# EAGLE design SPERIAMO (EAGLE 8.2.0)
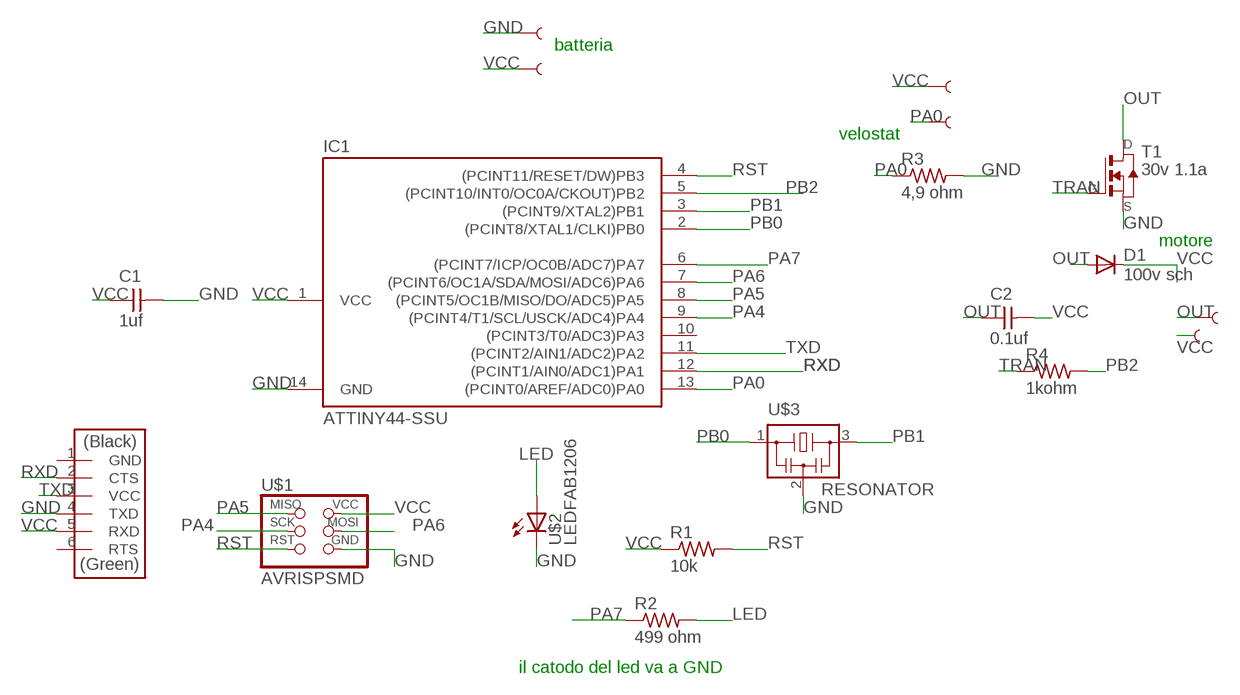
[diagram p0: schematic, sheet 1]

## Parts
C1  1uf  CAP-UNPOLARIZEDFAB  [C1206FAB]
C2  0.1uf  CAP-UNPOLARIZEDFAB  [C1206FAB]
D1  100v sch  DIODESOD123  [SOD123]
IC1  ATTINY44-SSU  [SOIC14]
R1  10k  RES-US1206FAB  [R1206FAB]
R2  499 ohm  RES-US1206FAB  [R1206FAB]
R3  4,9 ohm  RES-US1206FAB  [R1206FAB]
R4  1kohm  RES-US1206FAB  [R1206FAB]
T1  30v 1.1a  NMOSFETSOT23  [SOT-23]
U$1  AVRISPSMD  [2X03SMD]
U$2  LEDFAB1206  [LED1206FAB]
U$3  RESONATOR  [EFOBM]
U$4  FTDI-SMD-HEADER  [1X06SMD]
U$5  SEWTAP2  [PETAL-LONG-2]
U$6  SEWTAP2  [PETAL-LONG-2]
U$7  SEWTAP6  [PETAL-SMALL-2SIDE]
U$8  SEWTAP6  [PETAL-SMALL-2SIDE]
U$9  SEWTAP4  [PETAL-SMALL]
U$10  SEWTAP4  [PETAL-SMALL]

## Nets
GND: C1.2 IC1.14(GND) R3.2 T1.2(S) U$1.6(GND) U$2.2(C) U$3.2 U$4.4(TXD) U$10.1
LED: R2.2 U$2.1(A)
OUT: C2.1 D1.ANODE(A) T1.1(D) U$7.1
PA0: IC1.13((PCINT0/AREF/ADC0)PA0) R3.1 U$6.1
PA4: IC1.9((PCINT4/T1/SCL/USCK/ADC4)PA4) U$1.3(SCK)
PA5: IC1.8((PCINT5/OC1B/MISO/DO/ADC5)PA5) U$1.1(MISO)
PA6: IC1.7((PCINT6/OC1A/SDA/MOSI/ADC6)PA6) U$1.4(MOSI)
PA7: IC1.6((PCINT7/ICP/OC0B/ADC7)PA7) R2.1
PB0: IC1.2((PCINT8/XTAL1/CLKI)PB0) U$3.1
PB1: IC1.3((PCINT9/XTAL2)PB1) U$3.3
PB2: IC1.5((PCINT10/INT0/OC0A/CKOUT)PB2) R4.2
RST: IC1.4((PCINT11/RESET/DW)PB3) R1.2 U$1.5(RST)
RXD: IC1.12((PCINT1/AIN0/ADC1)PA1) U$4.2(CTS)
TRAN: R4.1 T1.3(G)
TXD: IC1.11((PCINT2/AIN1/ADC2)PA2) U$4.3(VCC)
VCC: C1.1 C2.2 D1.CATHODE(C) IC1.1(VCC) R1.1 U$1.2(VCC) U$4.5(RXD) U$5.1 U$8.1 U$9.1
Unconnected: IC1.10((PCINT3/T0/ADC3)PA3) U$4.1(GND) U$4.6(RTS)

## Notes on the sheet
- batteria
- velostat
- motore
- il catodo del led va a GND

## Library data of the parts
C1 C2 = 00_fab:CAP-UNPOLARIZED
D1 = 00_fab:DIODE: DIODE
IC1 = 00_fab:ATTINY44
R1-R4 = 00_fab:RES-US: Resistor (US Symbol)
T1 = 00_fab:NMOSFET: MOS FET
U$1 = 00_fab:AVRISP
U$2 = 00_fab:LED: LED
U$3 = 00_fab:RESONATOR
U$4 = 00_fab:FTDI-SMD-HEADER
U$5-U$10 = LilyPad-Wearables:SEWTAP

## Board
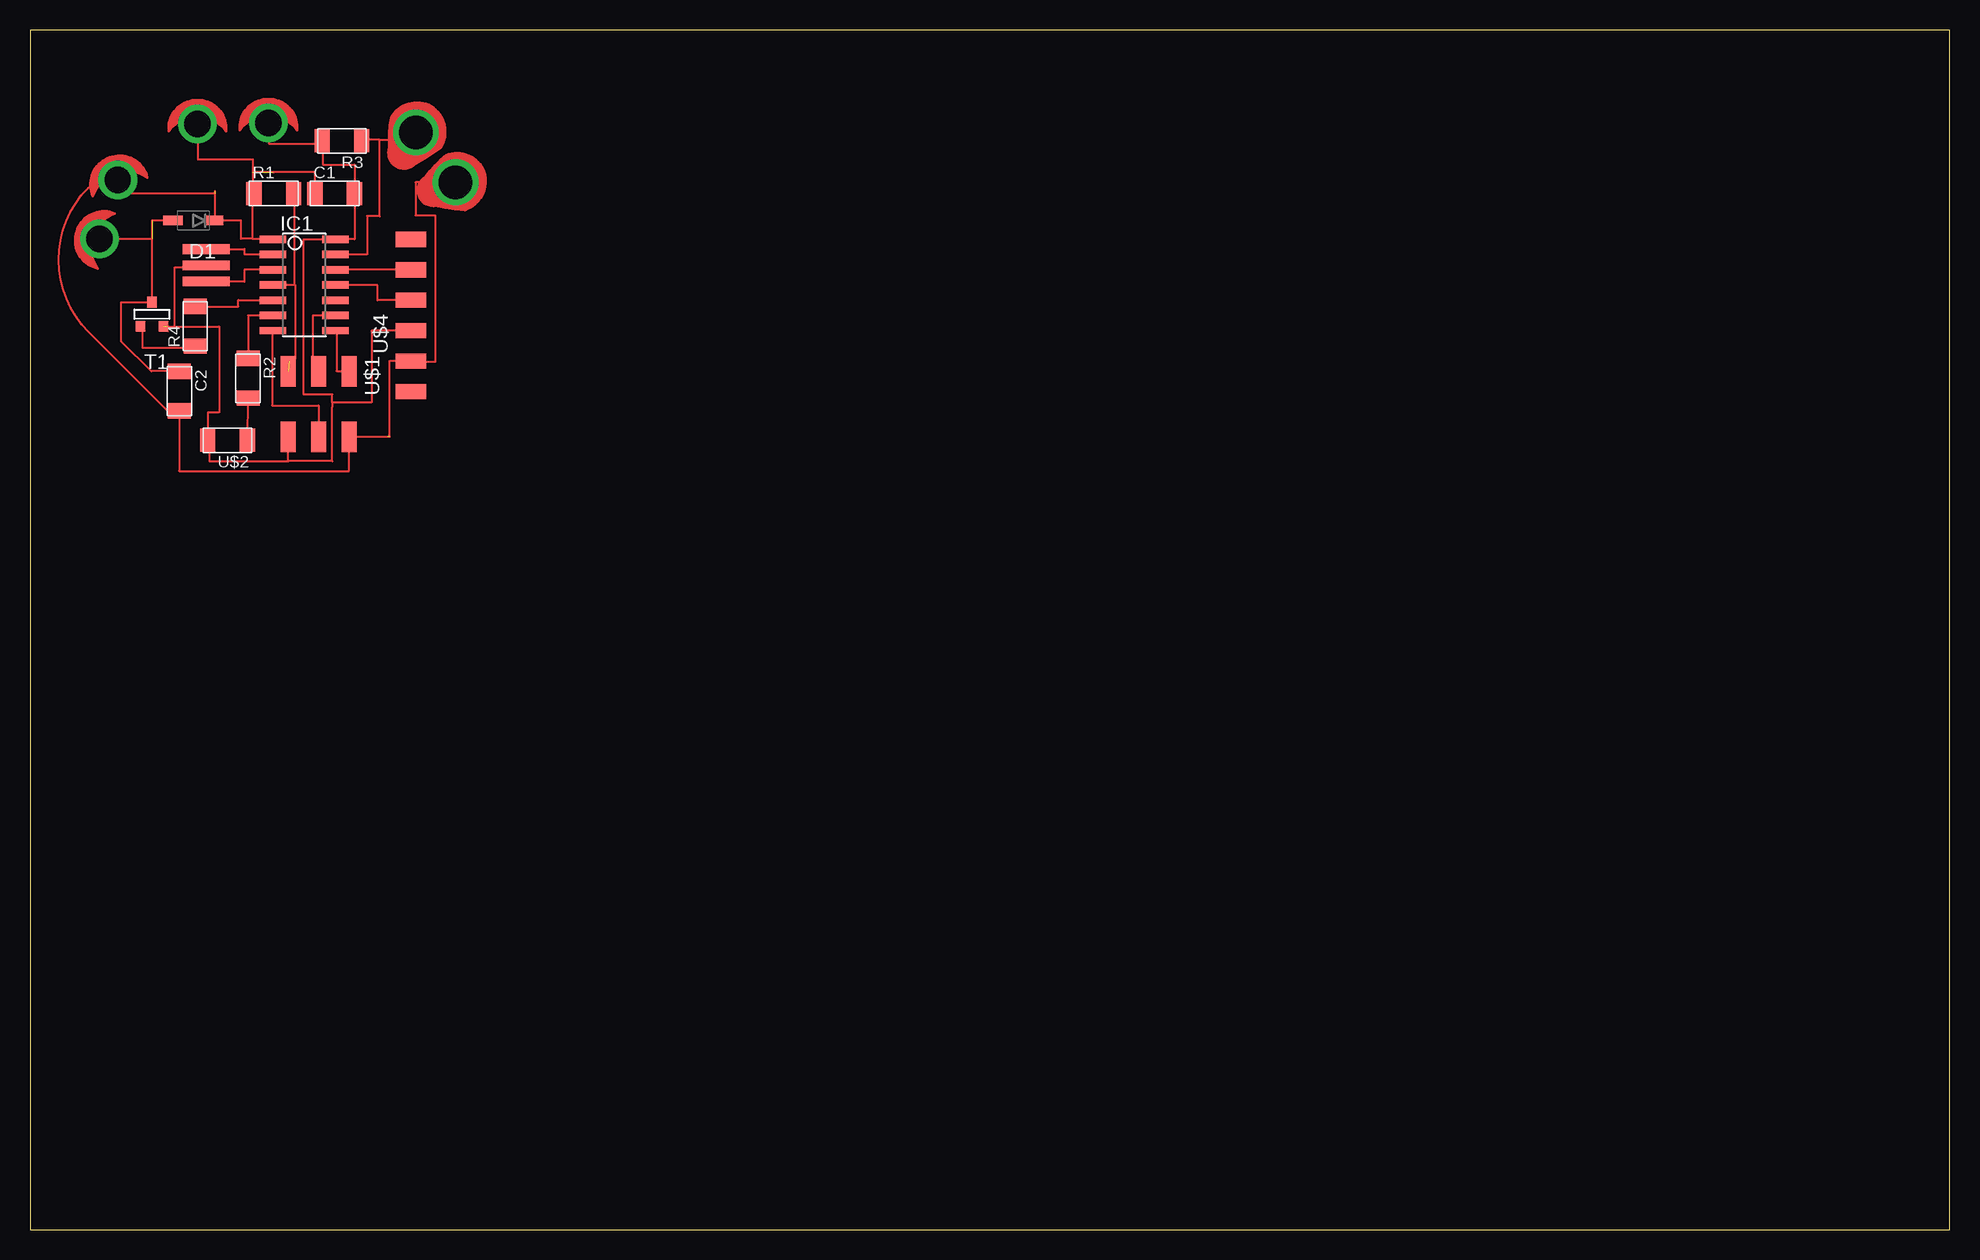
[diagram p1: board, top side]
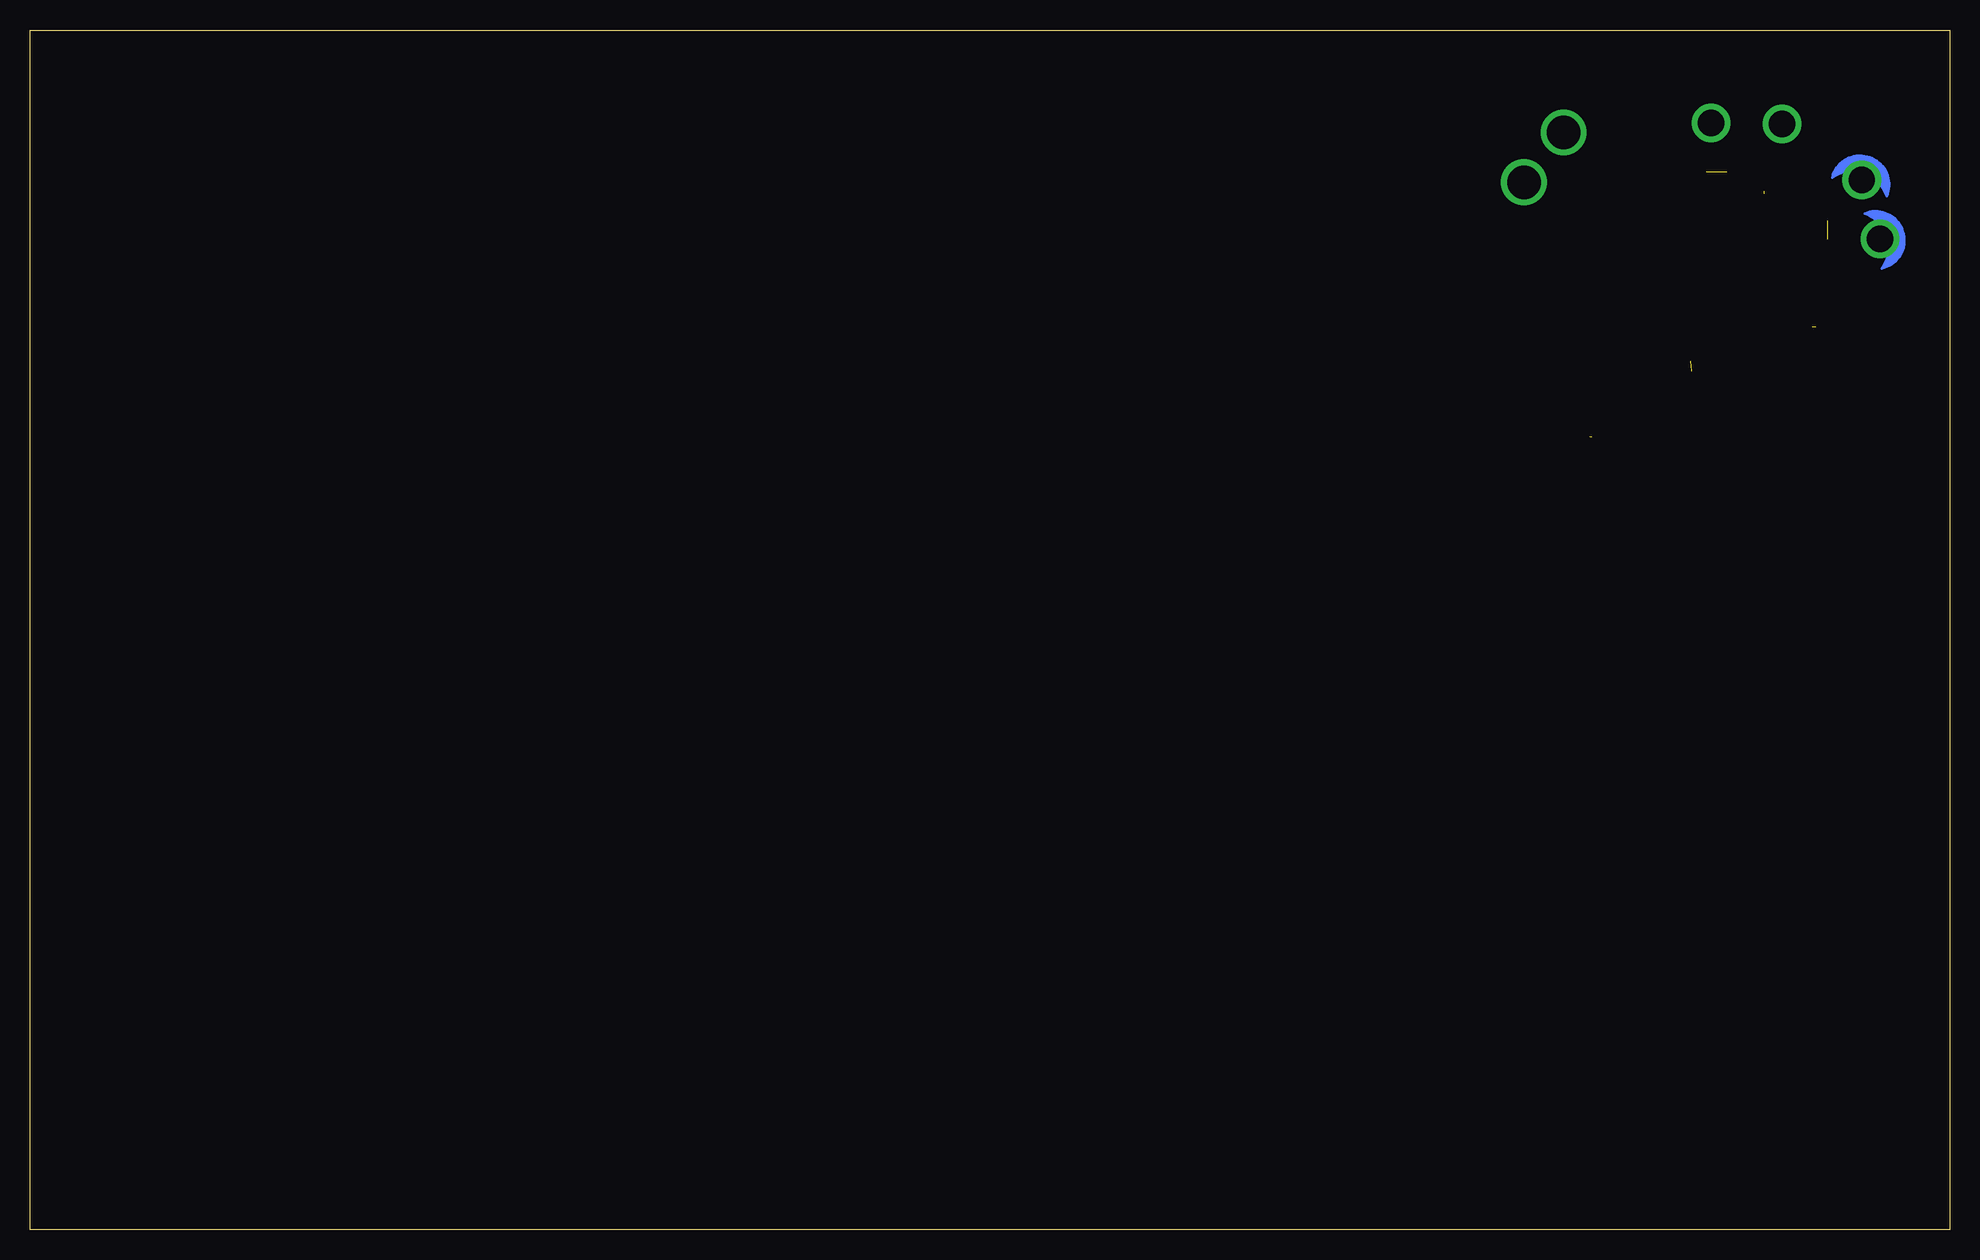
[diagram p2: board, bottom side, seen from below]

Size 160 x 100 mm. Coordinates in mm from the lower left corner, seen from the top.
Outline: 0,0 160,0 160,100 0,100 0,0
Copper layers (1*16): Top 0.035mm / dielectric 1.5mm / Bottom 0.035mm
Design rules "default *": minimum track width 16mil, minimum drill 0.35mm, track to track 16mil, track to pad 16mil, pad to pad 16mil, via to via 16mil, smd to smd 16mil, copper to edge 16mil, drill to drill 16mil, minimum pad ring 10mil, minimum via ring 8mil, stop-mask expansion 4mil, vias tented up to drill 0mil, thermal gap 10mil

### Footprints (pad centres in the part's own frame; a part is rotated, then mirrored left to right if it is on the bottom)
C1206FAB = smd 1.27 x 1.905: 1 -1.651,0; 2 1.651,0
SOD123 = smd 1.6 x 0.8: ANODE 1.7,0; CATHODE -1.7,0
SOIC14 = smd 0.61 x 2.21: 1 -3.81,-2.603; 2 -2.54,-2.603; 3 -1.27,-2.603; 4 0,-2.603; 5 1.27,-2.603; 6 2.54,-2.603; 7 3.81,-2.603; 8 3.81,2.603; 9 2.54,2.603; 10 1.27,2.603; 11 0,2.603; 12 -1.27,2.603; 13 -2.54,2.603; 14 -3.81,2.603
R1206FAB = smd 1.27 x 1.905: 1 -1.651,0; 2 1.651,0
SOT-23 = smd 0.787 x 0.889: 1 0.025,-1.016; 2 -0.94,1.016; 3 0.991,1.016
2X03SMD = smd 2.54 x 1.27: 1 -2.54,2.54; 2 2.92,2.54; 3 -2.54,0; 4 2.92,0; 5 -2.54,-2.54; 6 2.92,-2.54
LED1206FAB = smd 1.27 x 1.905: 1 -1.651,0; 2 1.651,0
EFOBM = smd 0.8 x 3.9: 1 -1.35,0; 2 0,0; 3 1.35,0
1X06SMD = smd 2.54 x 1.27: 1 0,6.35; 2 0,3.81; 3 0,1.27; 4 0,-1.27; 5 0,-3.81; 6 0,-6.35
PETAL-LONG-2 = drill 2.794: 1 0,0
PETAL-SMALL-2SIDE = drill 2.2: 1 0,0
PETAL-SMALL = drill 2.2: 1 0,0

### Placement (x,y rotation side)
C1  25.4,86.36 0 top
C2  12.45,69.9 270 top
D1  13.61,84.11 180 top
IC1  22.86,78.74 270 top
R1  20.32,86.36 0 top
R2  18.17,70.97 270 top
R3  26,90.76 180 top
R4  13.77,75.3 90 top
T1  10.2,76.3 179.7 top
U$1  24.06,69.02 270 top
U$2  16.47,65.8 180 top
U$3  14.68,80.38 270 top
U$4  31.75,76.2 0 top
U$5  35.47,87.3 109.9 top
U$6  32.16,91.45 149.9 top
U$7  5.79,82.59 252.8 top
U$8  7.32,87.49 199.1 top
U$9  13.96,92.16 180 top
U$10  19.87,92.25 180 top

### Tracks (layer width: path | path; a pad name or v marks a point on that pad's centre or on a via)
GND  (1 unrouted)
  Top 0.152: U$2.2 14.95,65.8 14.95,64.05 21.52,64.05 | 21.52,64.05 | 21.52,64.05 U$1.6 | 21.52,64.05 25.2,64.05 25.2,68.58 25.2,68.94 | 25.2,68.94 25.2,69.61 22.81,69.61 22.81,82.55 IC1.14 27.05,82.55 C1.2 27.05,88.77 24.4,88.77 24.4,90.53 | U$4.4 28.47,74.93 28.47,68.94 25.2,68.94 | U$2.2 15.24,65.8 15.24,66.04 14.88,65.69 14.88,65.35 14.81,65.42 U$2.2 | R3.2 24.4,90.76 24.4,90.53 | U$10.1 19.91,92.25 19.91,90.53 24.4,90.53 | T1.2 12.06,75.28 12.06,80.22 14.68,80.22 U$3.2 | 11.43,75.28 15.76,75.28 15.76,68.12 14.81,68.12 U$2.2
LED
  Top 0.152: U$2.1 18.14,65.8 R2.2
OUT  (1 unrouted)
  Top 0.152: 11.43,83.82 11.43,83.96 12.03,83.96 12.03,84.11 D1.ANODE 10.18,84.11 T1.1 7.58,77.3 7.58,74.04 7.62,74.04 10.11,71.55 C2.1 | 10.18,82.55 5.79,82.55 U$7.1
PA0
  Top 0.152: IC1.13 28.1,81.28 28.1,84.5 28.12,84.5 29.16,84.48 29.14,90.84 | 30.64,93.05 U$6.1 | 29.14,90.84 27.65,90.86 R3.1 | 29.14,90.84 32.16,90.86 U$6.1 | U$6.1 31.75,91.44
PA4
  Top 0.152: U$1.3 24.06,72.54 23.58,72.54 23.58,76.2 IC1.9
PA5
  Top 0.152: 25.4,74.93 IC1.8 25.54,74.93 25.54,71.56 U$1.1
PA6
  Top 0.152: 20.32,74.93 IC1.7 20.18,74.93 20.18,68.69 24.06,68.69 U$1.4
PA7
  Top 0.152: IC1.6 18.17,76.2 R2.1
PB0
  Top 0.152: IC1.2 17.88,81.28 17.88,81.75 15.24,81.75 | 15.24,81.75 14.68,81.75 U$3.1 15.24,81.73 15.24,81.75
PB1
  Top 0.152: IC1.3 17.86,80.01 17.86,79 14.68,79 U$3.3
PB2
  Top 0.152: IC1.5 20.26,77.41 | 20.26,77.55 IC1.5 | R4.2 17.36,76.95 17.36,77.49 20.26,77.49 IC1.5
RST  (1 unrouted)
  Top 0.152: 22.08,78.74 21.79,78.73 20.92,78.73 20.92,78.69 20.26,78.69 IC1.4 | 22.08,78.74 22.09,78.76 22.09,78.74 | 22.09,78.74 22.09,72.55 21.59,72.57 21.59,72.39 | 21.59,86.36 R1.2 22.08,86.36 22.08,78.74 | 22.09,78.74 22.08,78.74
RXD
  Top 0.152: U$4.2 IC1.12
TRAN
  Top 0.152: T1.3 9.37,75.29 9.37,73.51 13.77,73.51 R4.1
TXD
  Top 0.152: U$4.3 28.97,77.47 28.97,78.72 25.46,78.72 IC1.11
VCC  (3 unrouted)
  Top 0.152: 18.53,82.59 18.53,86.36 R1.1 18.58,86.36 18.58,88.13 | 18.53,82.59 20.26,82.59 IC1.1 20.32,82.55 | 18.58,88.13 23.75,88.13 C1.1 | 18.53,82.59 17.6,82.59 17.6,84.12 15.31,84.12 D1.CATHODE 15.43,84.11 15.43,86.57 | 29.81,66.1 U$1.2 26.6,63.25 12.43,63.25 12.43,68.24 C2.2 11.47,68.24 4.89,74.83 arc-101 6.11,87.9 arc-106 U$8.1 8.44,86.36 15.43,86.36 | 20.32,88.13 20.26,88.13 20.32,88.13 | 29.21,66.1 29.99,66.1 29.99,72.43 31.75,72.43 U$4.5 | U$4.5 31.7,72.39 31.7,72.31 31.75,72.31 | U$5.1 32.15,87.31 32.15,84.55 33.79,84.55 33.79,72.31 31.75,72.31 | 31.75,72.31 U$4.5 | U$9.1 13.99,92.16 13.99,89.21 18.58,89.21 18.58,88.13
